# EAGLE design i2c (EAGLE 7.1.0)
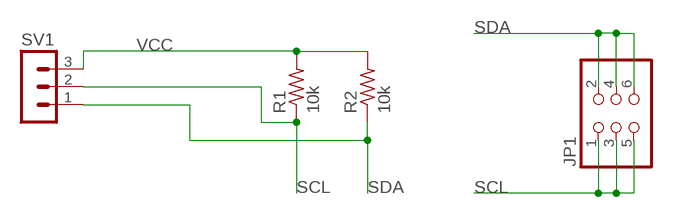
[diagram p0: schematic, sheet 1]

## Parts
JP1  PINHD-2X3-SMD  [2X03SMD]
R1  10k  RESISTOR1206  [1206]
R2  10k  RESISTOR1206  [1206]
SV1  MA03-1  [MA03-1]

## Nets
SCL: JP1.1 JP1.3 JP1.5 R1.1 SV1.2
SDA: JP1.2 JP1.4 JP1.6 R2.1 SV1.1
VCC: R1.2 R2.2 SV1.3

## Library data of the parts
JP1 = 01_FAB_Hello:PINHD-2X3-SMD: PIN HEADER
R1 R2 = 01_FAB_Hello:RESISTOR
SV1 = con-lstb:MA03-1: PIN HEADER; OC_FARNELL: unknown; OC_NEWARK: unknown

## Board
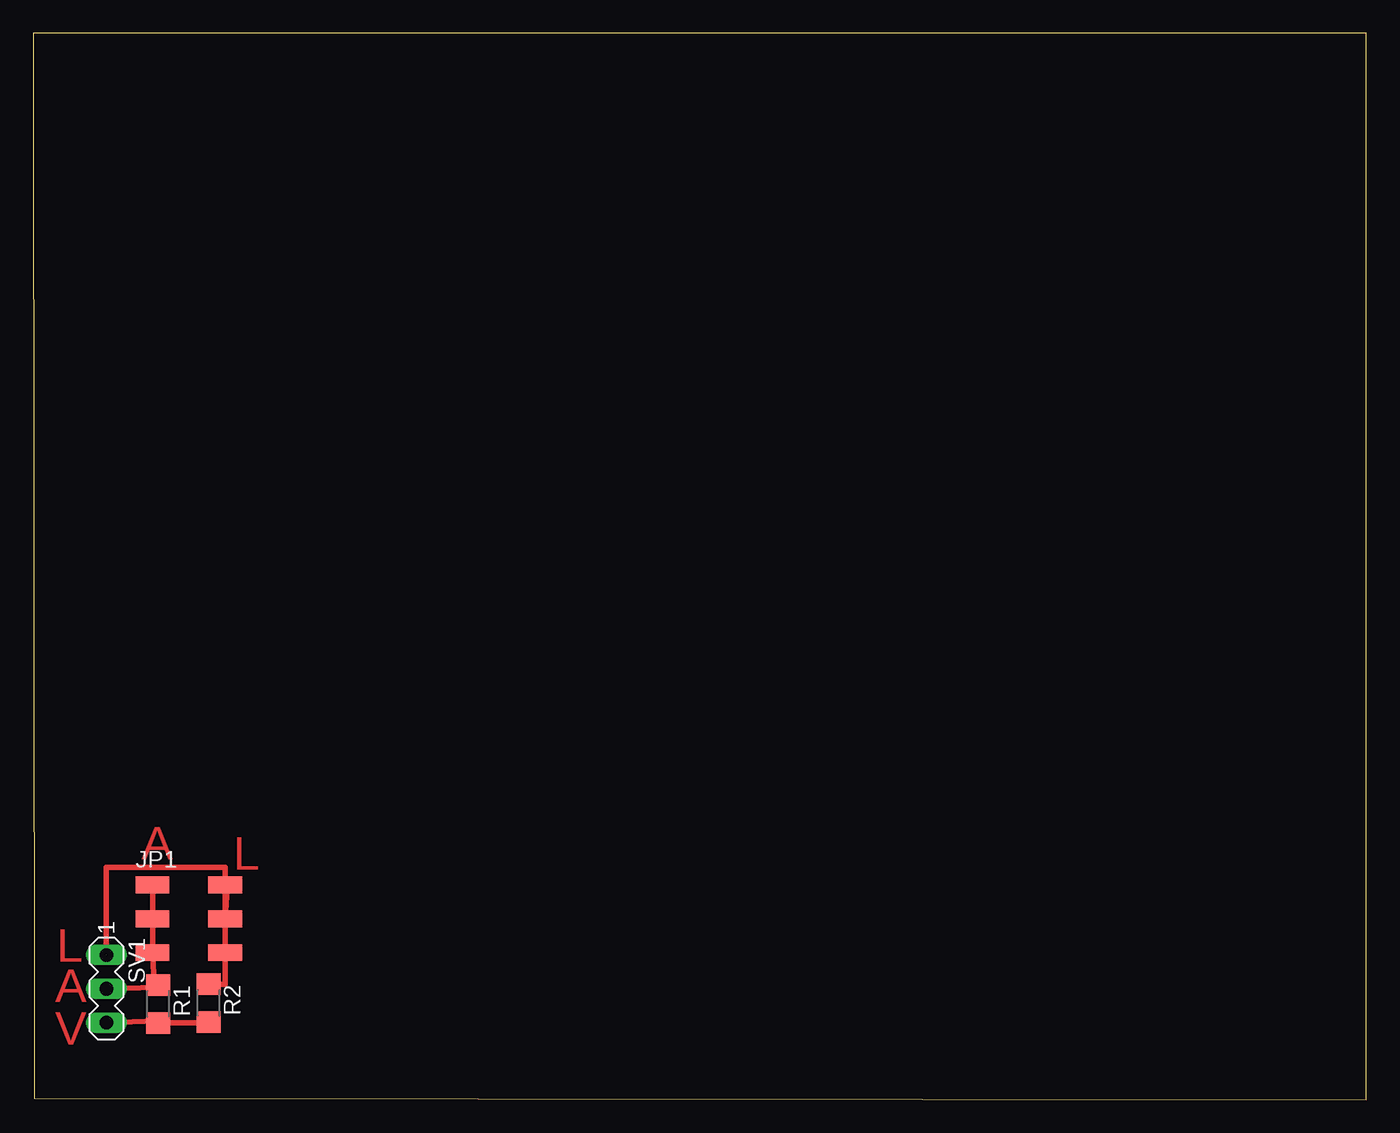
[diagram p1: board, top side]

Size 100 x 80 mm. Coordinates in mm from the lower left corner, seen from the top.
Outline: 0.08,0.08 100,0 100,80 0,80 0.08,0.08
Copper layers (1*16): Top 0.035mm / dielectric 1.5mm / Bottom 0.035mm
Design rules "default": minimum track width 15mil, minimum drill 24mil, track to track 15mil, track to pad 15mil, pad to pad 15mil, via to via 15mil, smd to smd 15mil, copper to edge 40mil, drill to drill 8mil, minimum pad ring 10mil, minimum via ring 8mil, stop-mask expansion 4mil, vias tented up to drill 0mil, thermal gap 10mil

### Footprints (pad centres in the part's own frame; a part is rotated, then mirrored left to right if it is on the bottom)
2X03SMD = smd 2.54 x 1.27: 1 -2.54,2.54; 2 2.92,2.54; 3 -2.54,0; 4 2.92,0; 5 -2.54,-2.54; 6 2.92,-2.54
1206 = smd 1.6 x 1.803: 1 -1.422,0; 2 1.422,0
MA03-1 = drill 1.016 long: 1 -2.54,0; 2 0,0; 3 2.54,0

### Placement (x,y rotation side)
JP1  11.48,13.56 0 top
R1  9.37,7.16 270 top
R2  13.16,7.24 270 top
SV1  5.49,8.31 270 top

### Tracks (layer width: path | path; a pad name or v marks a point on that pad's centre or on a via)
SCL
  Top 0.406: SV1.2 9.37,8.43 R1.1 9.07,8.59 JP1.5 JP1.3 JP1.1
SDA  (1 unrouted)
  Top 0.406: 5.46,10.85 5.46,17.42 14.4,17.42 JP1.2 JP1.4 14.53,15.8 14.38,15.8 14.38,12.65 JP1.6 14.4,8.66 R2.1
VCC
  Top 0.406: SV1.3 9.37,5.89 R1.2 13.16,5.74 R2.2

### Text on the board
Top: A | L | L | A | V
